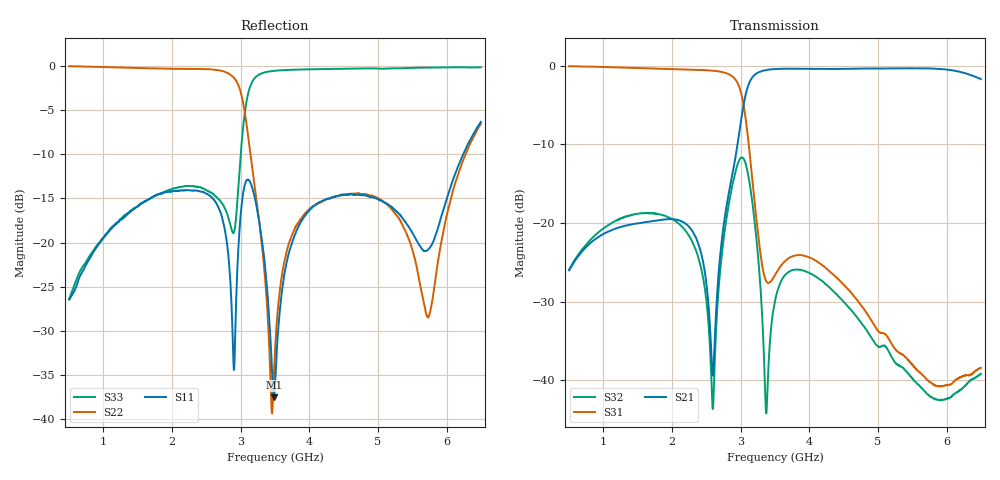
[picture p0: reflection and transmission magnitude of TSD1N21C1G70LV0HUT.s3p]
# MHZ S RI R 50
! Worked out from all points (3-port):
!   1201 points, 500 MHz to 6.5 GHz, reference 50 ohm
!   strongest paths, dB at 500 MHz, 2 GHz, 3.5 GHz, 5 GHz, 6.5 GHz:
!     S21: -26.0, -19.5, -0.4, -0.3, -1.7
!     S31: -0.1, -0.4, -26.6, -33.6, -38.4
!     S32: -25.9, -19.5, -29.9, -35.7, -39.2
!   lowest |S11| = -37.5 dB at 3.485 GHz (marker M1), VSWR 1.03, Z = 50.9 - j1 ohm
!   |S11| at or under -10 dB: start of sweep to 6.242 GHz
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500  -0.0252 -0.0403  0.0139 0.048  0.937 -0.331
     0.014 0.0481  0.907 -0.417  0.0259 0.0435
     0.937 -0.331  0.0257 0.0436  -0.00218 -0.0478
2090  -0.0104 0.197  0.0693 0.0782  -0.0791 -0.946
      0.0695 0.0781  -0.198 -0.944  0.0615 -0.0788
      -0.0785 -0.946  0.0614 -0.0787  -0.0337 -0.203
2595  0.177 -0.00458  -0.00351 0.01  -0.701 -0.612
      -0.0036 0.0101  -0.665 -0.687  0.00604 -0.00251
      -0.7 -0.612  0.00608 -0.0025  -0.000431 -0.189
2990  0.082 0.0995  -0.4 0.0586  -0.548 0.45
      -0.4 0.0579  -0.703 0.213  0.141 -0.212
      -0.548 0.449  0.141 -0.214  0.278 0.036
3370  -0.0199 -0.0606  0.00919 0.938  -0.037 0.0215
      0.00903 0.939  -0.0349 0.0395  0.00171 0.0061
      -0.0371 0.0215  0.00173 0.00595  0.399 -0.834
3485  0.00893 -0.00984  0.236 0.921  -0.0451 -0.00598
      0.235 0.922  -0.002 -0.0178  0.0257 -0.0148
      -0.0451 -0.00611  0.0256 -0.0149  0.246 -0.907
3500  0.0144 -0.00573  0.262 0.915  -0.046 -0.00845
      0.261 0.916  0.000821 -0.0246  0.0268 -0.0175
      -0.046 -0.00855  0.0268 -0.0176  0.229 -0.913
4900  0.114 -0.141  0.946 -0.145  -0.0241 -0.00194
      0.95 -0.145  -0.15 -0.107  -0.0162 -0.00978
      -0.0241 -0.002  -0.0161 -0.00973  -0.728 -0.641
5730  0.0888 -0.0202  0.645 -0.713  -0.00754 0.00653
      0.644 -0.714  -0.00277 0.0375  -0.00815 -0.00085
      -0.00754 0.00653  -0.00807 -0.000819  -0.908 -0.369
6500  0.473 0.0967  -0.0691 -0.821  0.000706 0.0119
      -0.0726 -0.819  0.394 -0.257  -0.0113 0.00072
      0.00051 0.012  -0.011 0.000599  -0.946 -0.275
